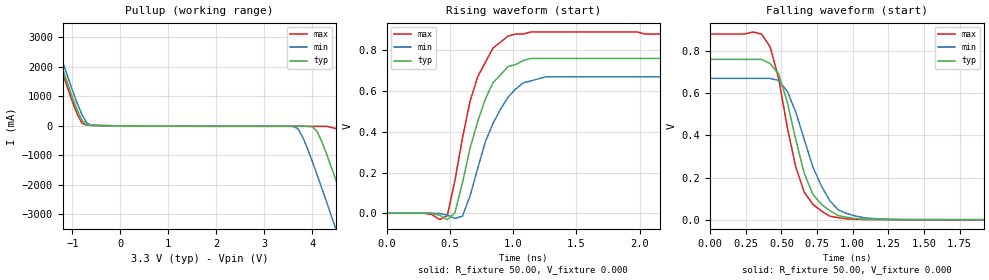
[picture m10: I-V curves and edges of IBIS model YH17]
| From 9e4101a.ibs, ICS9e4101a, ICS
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|   Model YH17
[Model]   YH17
Model_type   Open_source
Polarity   Inverting
C_comp   5.50pF   5.00pF   6.00pF
[Temperature Range]   27.00   70.00   0.000
[Voltage Range]   3.30V   3.00V   3.70V
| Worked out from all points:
|   slope of the pullup table from 0 to 0.495 V, typ, clamps not added: 56.2 ohm
|   rising waveform, R_fixture 50.00, V_fixture 0.000: 20-80 % time 215ps typ, 244ps min, 205ps max; typ from 0 V to 0.76 V
|   falling waveform, R_fixture 50.00, V_fixture 0.000: 20-80 % time 183ps typ, 218ps min, 171ps max; typ from 0.76 V to 0 V
[Pullup]
| voltage   I(typ)   I(min)   I(max)
-3.3V     12.3A      12.52A     12.16A
-1.7V     4.31A      4.55A      4.16A
-1.5V     3.33A      3.58A      3.17A
-900mV    540mA      770mA      400mA
-700mV    28.62mA    98.17mA    20.44mA
3.7V      -15.27mA   -98.55mA   -17.78mA
4.1V      -190mA     -1.66A     -17.81mA
4.5V      -1.87A     -3.54A     -94.69mA
4.7V      -2.82A     -4.51A     -810mA
4.9V      -3.78A     -5.48A     -1.72A
5.3V      -5.73A     -7.43A     -3.63A
6.6V      -12.13A    -13.84A    -10.01A
[Ramp]
| variable   typ   min   max
dV/dt_r   0.46/0.21n   0.40/0.24n   0.53/0.20n
dV/dt_f   0.45/0.18n   0.40/0.21n   0.53/0.16n
R_load = 50.00
[Rising Waveform]
R_fixture = 50.00
V_fixture = 0.000
V_fixture_min = 0.000
V_fixture_max = 0.000
| time   V(typ)   V(min)   V(max)
0s        0V         0V         0V
480ps     -31.45mV   -8.81mV    -11.53mV
540ps     2.33mV     -25.49mV   160mV
600ps     150mV      -13.74mV   370mV
720ps     450mV      220mV      670mV
840ps     640mV      440mV      810mV
960ps     720mV      570mV      870mV
1.08ns    750mV      640mV      880mV
1.26ns    760mV      670mV      890mV
3ns       760mV      670mV      880mV
[Falling Waveform]
R_fixture = 50.00
V_fixture = 0.000
V_fixture_min = 0.000
V_fixture_max = 0.000
| time   V(typ)   V(min)   V(max)
0s        760mV      670mV      880mV
300ps     760mV      670mV      890mV
420ps     740mV      670mV      820mV
480ps     690mV      660mV      670mV
540ps     560mV      610mV      440mV
660ps     220mV      380mV      130mV
720ps     120mV      250mV      72.97mV
840ps     42.69mV    89.32mV    16.24mV
1.2ns     1.01mV     2.93mV     290uV
3ns       3.96uV     0V         1.45uV
